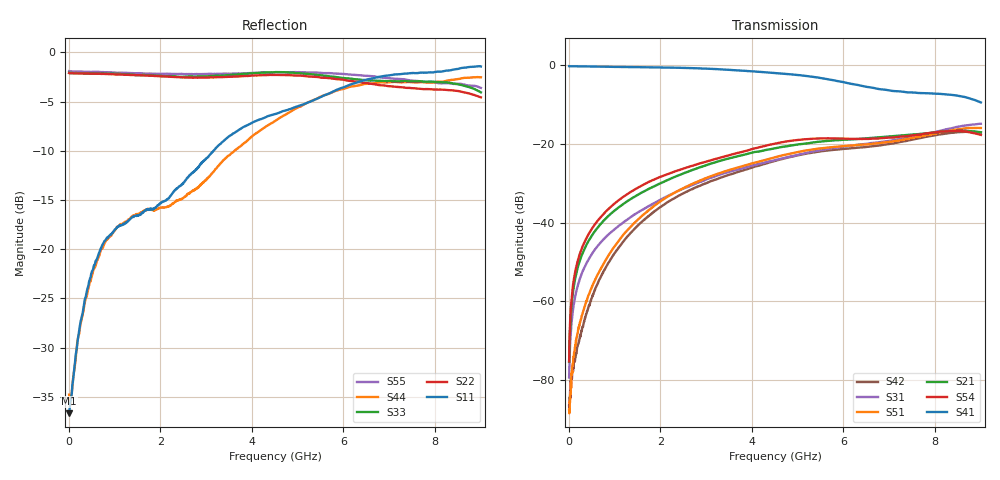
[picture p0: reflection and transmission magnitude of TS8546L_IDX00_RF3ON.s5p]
# GHz S DB R 50
! CMT, SN0916, 25263762, 26.7.0
! Date: 16.07.2026 08:29:44
! Data: Format
! Freq S1.1:dB/Ang S1.2:dB/Ang S1.3:dB/Ang S1.4:dB/Ang S1.5:dB/Ang
!  S2.1:dB/Ang S2.2:dB/Ang S2.3:dB/Ang S2.4:dB/Ang S2.5:dB/Ang
!  S3.1:dB/Ang S3.2:dB/Ang S3.3:dB/Ang S3.4:dB/Ang S3.5:dB/Ang
!  S4.1:dB/Ang S4.2:dB/Ang S4.3:dB/Ang S4.4:dB/Ang S4.5:dB/Ang
!  S5.1:dB/Ang S5.2:dB/Ang S5.3:dB/Ang S5.4:dB/Ang S5.5:dB/Ang
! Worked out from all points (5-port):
!   2001 points, 10 MHz to 9 GHz, reference 50 ohm
!   strongest paths, dB at 10 MHz, 2.257 GHz, 4.505 GHz, 6.753 GHz, 9 GHz:
!     S41: -0.2, -0.6, -1.9, -6.0, -9.4
!     S54: -75.3, -27.2, -19.9, -18.6, -17.7
!     S21: -75.4, -28.6, -21.1, -18.3, -17.0
!     S51: -87.7, -32.7, -23.3, -19.8, -15.9
!     S31: -79.4, -32.7, -24.1, -19.6, -14.8
!     S42: -86.6, -34.1, -24.3, -20.4, -17.1
!   lowest |S11| = -36.7 dB at 10 MHz (marker M1), VSWR 1.03, Z = 51.5 - j0.0495 ohm
!   |S11| at or under -10 dB: start of sweep to 3.159 GHz
